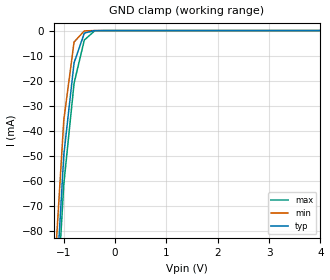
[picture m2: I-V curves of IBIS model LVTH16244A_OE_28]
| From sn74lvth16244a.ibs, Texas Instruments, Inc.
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|   Model LVTH16244A Input_OE_28
[Model]   LVTH16244A_OE_28
Model_type  Input
Polarity   Inverting
Vinl = 0.8V
Vinh = 2.0V
| variable   typ   min   max
C_comp   4pf   NA   NA
[Temperature Range]   40   -25   100
| Ambient temperature   25   -40   85
[Voltage range]   2.8   2.7   2.9
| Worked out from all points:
|   GND clamp passes 1 mA (typ) near -0.60 V on its own axis
[GND Clamp]
|   Voltage   I(typ)   I(min)   I(max)
-5V       -2.09A     -2.417A    -1.843A
-1.2V     -121.4mA   -103.3mA   -132.7mA
-1V       -49.81mA   -35.82mA   -61.52mA
-800mV    -12.93mA   -4.589mA   -21.1mA
-600mV    -1.008mA   -122uA     -3.782mA
-400mV    -5.028uA   -309.1nA   -141.4uA
-200mV    -4.054nA   -129.2nA   -417.2nA
5V        515pA      268.7nA    364pA
